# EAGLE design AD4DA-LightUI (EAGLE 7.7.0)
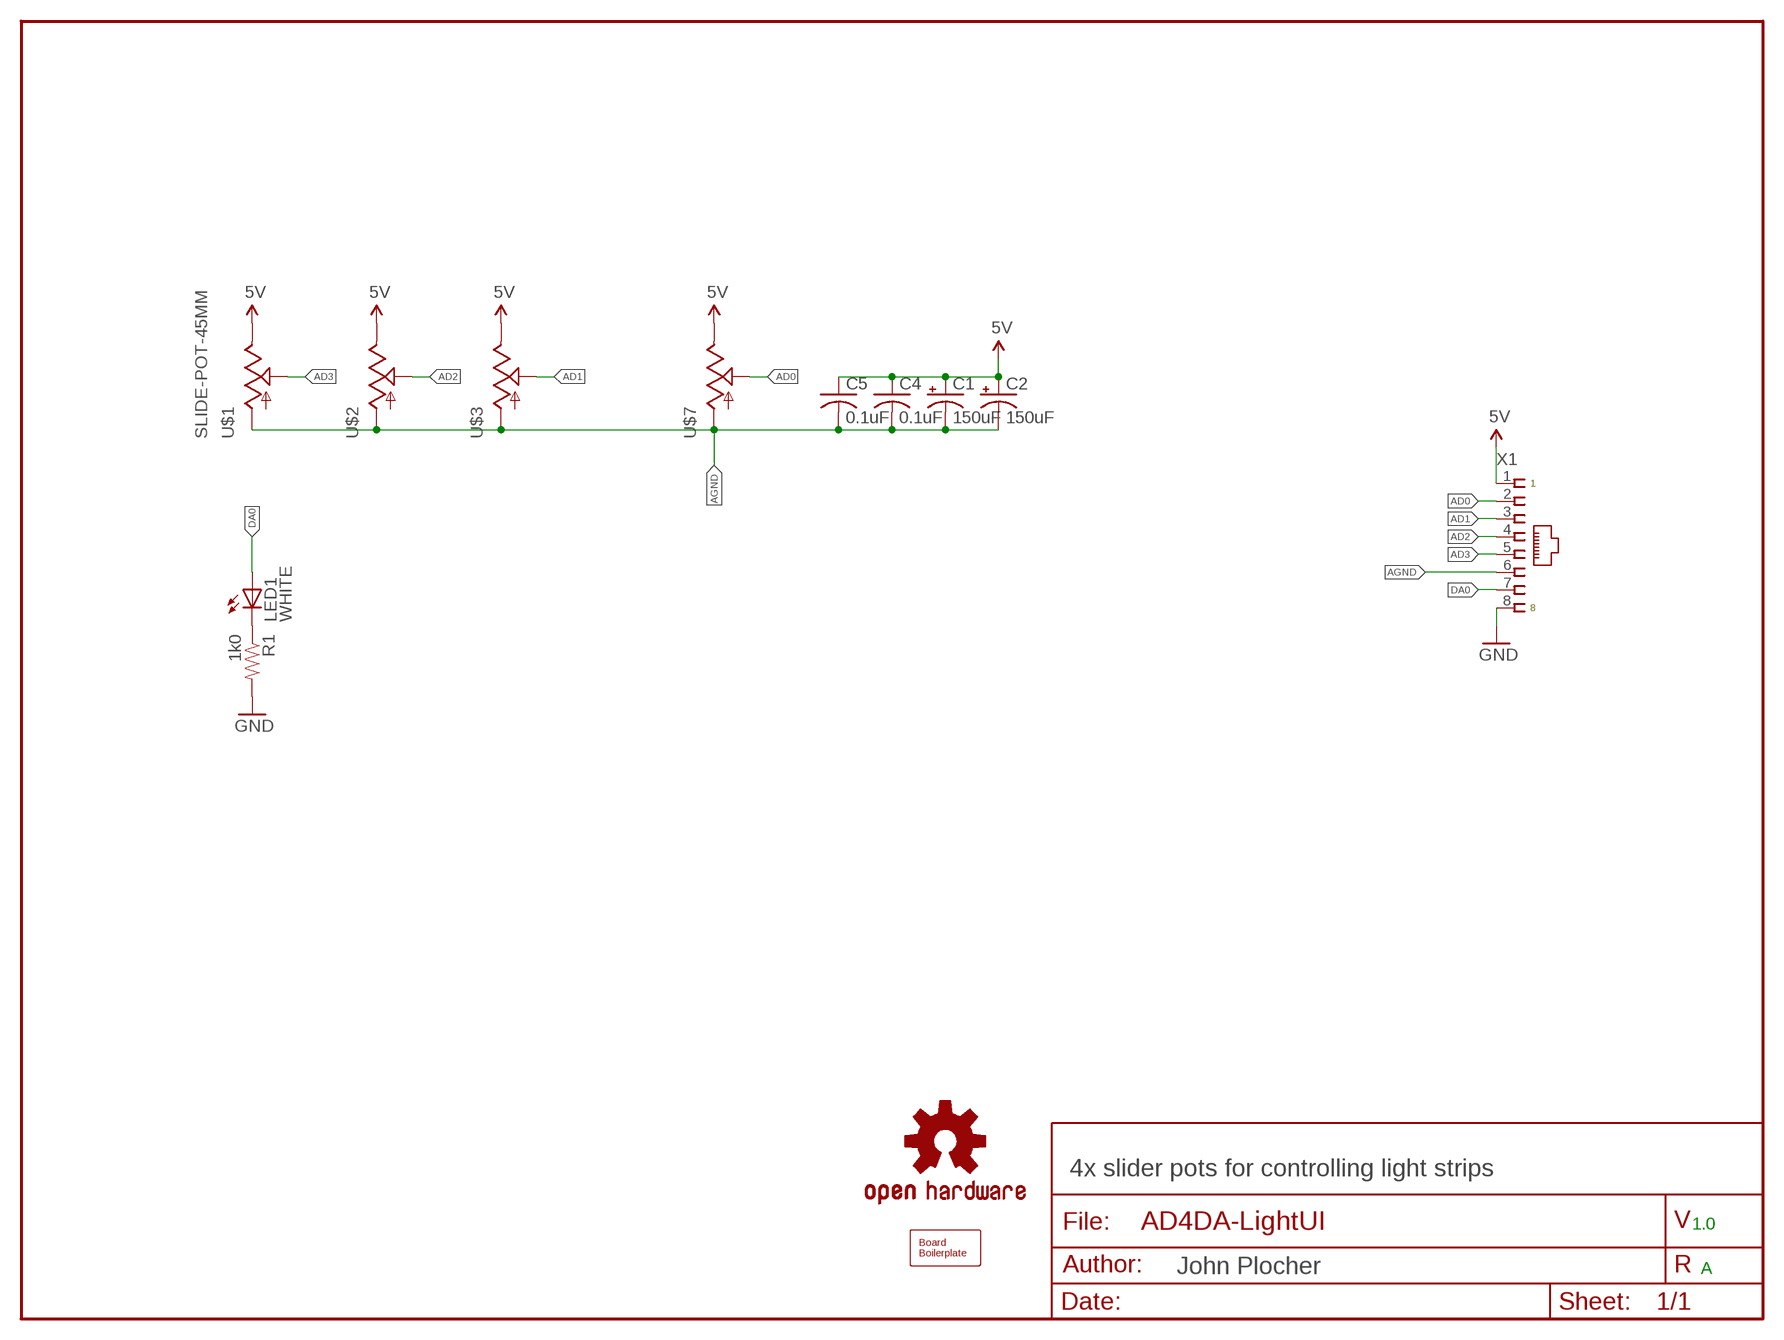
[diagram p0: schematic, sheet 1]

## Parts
C1  150uF  CAP-POLPTH-5MM  [E5-10.5]
C2  150uF  CAP-POLPTH-5MM  [E5-10.5]
C4  0.1uF  CAPPTH1  [C050-024X044]
C5  0.1uF  CAPPTH1  [C050-024X044]
LED1  WHITE  LEDLED5MM  [LED5MM]
LOGO1  DOC-OSHW-LOGO-L  [OSHW-LOGO-L]
R1  1k0  RPTH03  [AXIAL-0.3-RES]
U$1  SLIDE-POT-45MM  R-SLIDE-POT  [SLIDER-45MM-LARGE]
U$2  R-SLIDE-POT  [SLIDER-45MM-LARGE]
U$3  R-SLIDE-POT  [SLIDER-45MM-LARGE]
U$7  R-SLIDE-POT  [SLIDER-45MM-LARGE]
U$9  BOARD80X100  [BOARD-DINRAIL-3.17INX10CM]
X1  CONNECTOR-RJ45-FRONT  [RJ45-NO-SHIELD]

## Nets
5V: C1.+ C2.+ C4.1 C5.1 U$1.E U$2.E U$3.E U$7.E X1.1
AD0: U$7.S X1.2
AD1: U$3.S X1.3
AD2: U$2.S X1.4
AD3: U$1.S X1.5
AGND: C1.- C2.- C4.2 C5.2 U$1.A U$2.A U$3.A U$7.A X1.6
DA0: LED1.A X1.7
GND: R1.P$2 X1.8
N$2: LED1.K(C) R1.P$1
Unconnected: U$1.AGND@0(AGND) U$2.AGND@0(AGND) U$3.AGND@0(AGND) U$7.AGND@0(AGND)

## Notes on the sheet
- 4x slider pots for controlling light strips
- 1.0
- A

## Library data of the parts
C1 C2 = SPCoast:CAP-POL*
C4 C5 = SPCoast:CAP*
LED1 = SPCoast:LED*
LOGO1 = SPCoast:DOC-OSHW-LOGO-: Open Source Hardware Logo
R1 = SPCoast:R*: Resistor
U$1-U$3 U$7 = SPCoast:R-SLIDE-POT: Slide-type potentiometer- COM-9119
U$9 = SPCoast:BOARD
X1 = SPCoast:CONNECTOR-RJ45: Tyco CORCOM Modular RJ Jacks No Shield; AMP: 520151-4; OPL: none

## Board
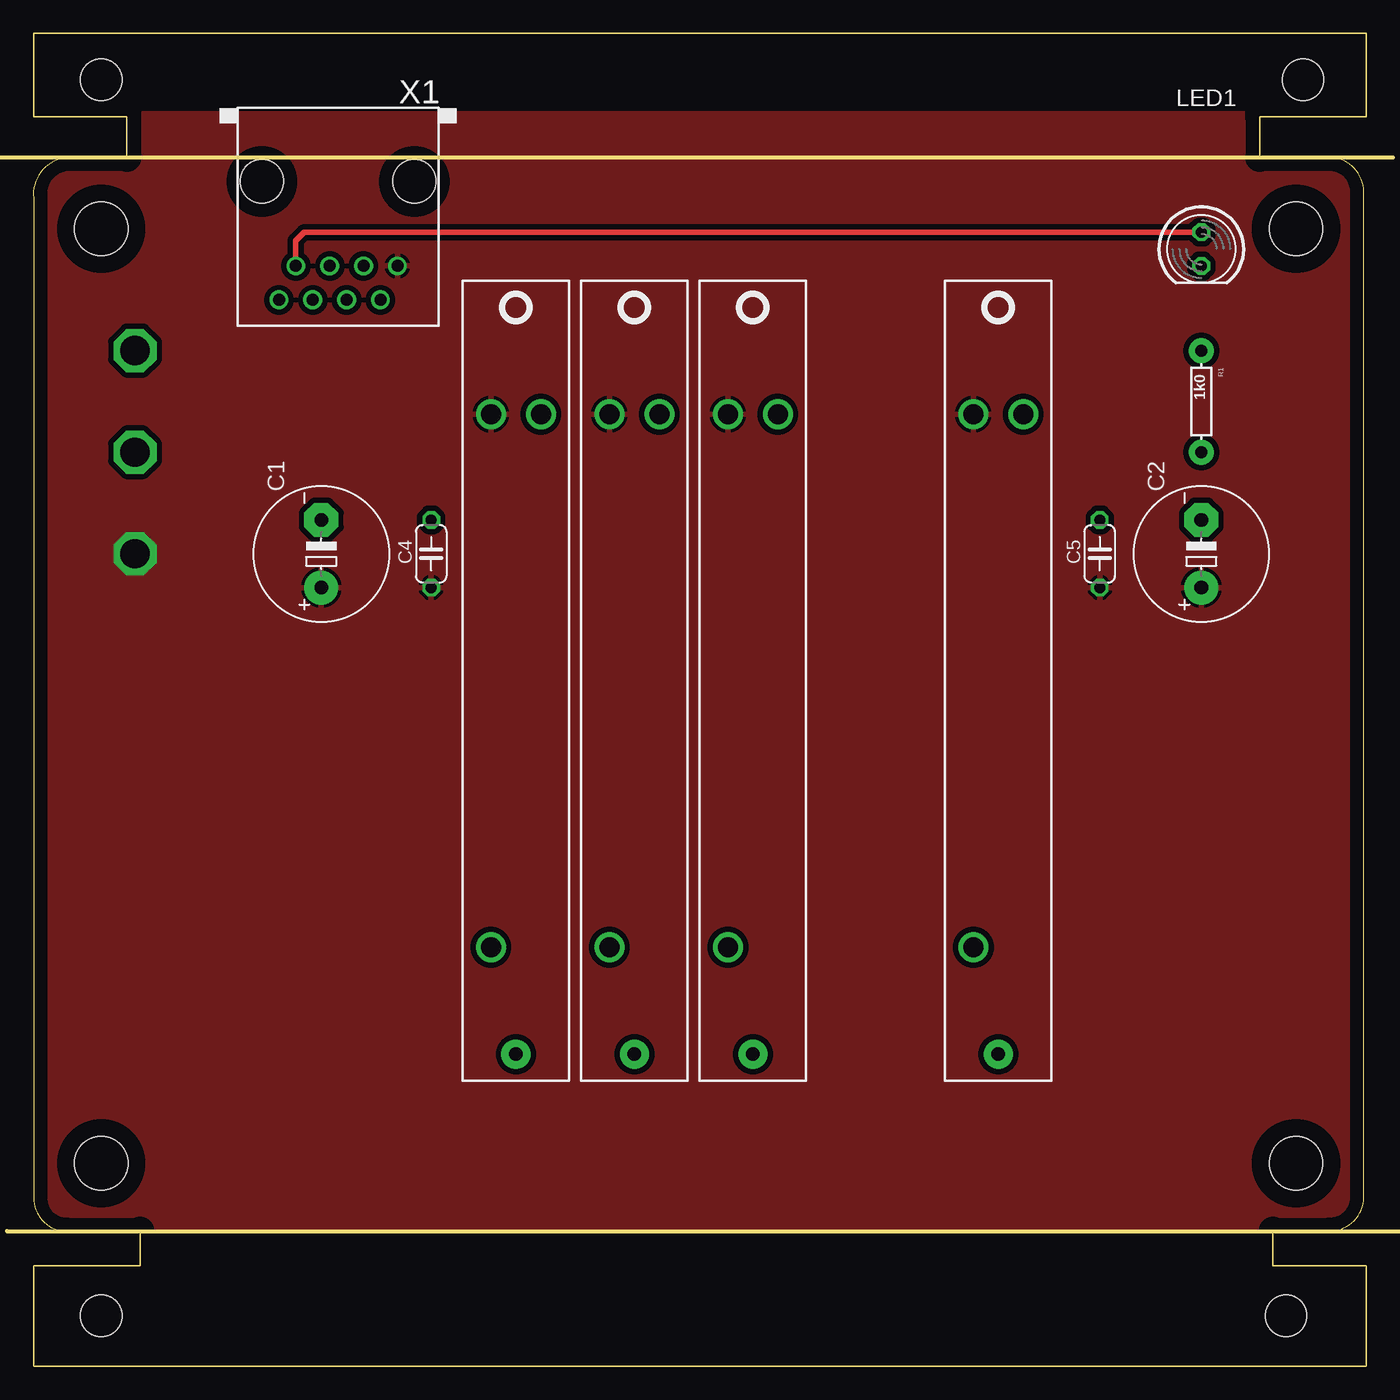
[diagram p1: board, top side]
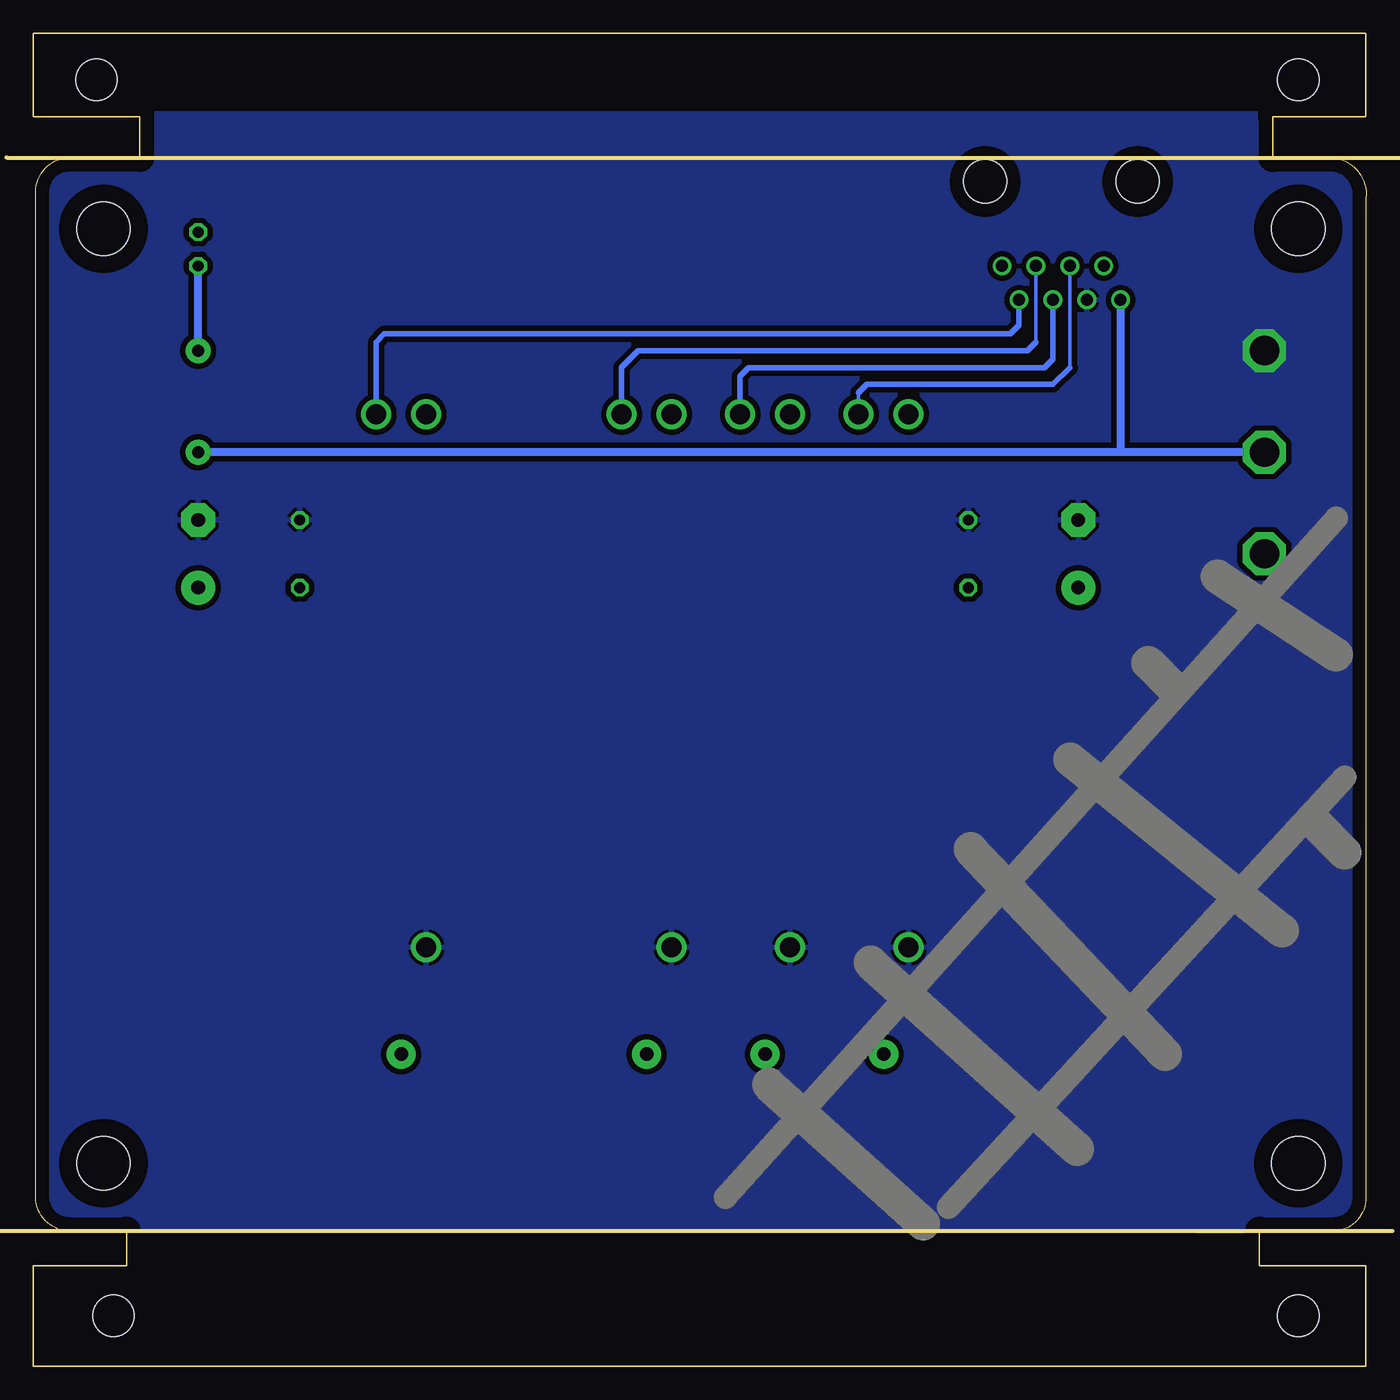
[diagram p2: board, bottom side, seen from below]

Size 100.01 x 100 mm. Coordinates in mm from the lower left corner, seen from the top.
Copper layers (1*16): Top 0.035mm / dielectric 1.5mm / Bottom 0.035mm
Design rules "default": minimum track width 10mil, minimum drill 0.6mm, track to track 8mil, track to pad 8mil, pad to pad 8mil, via to via 8mil, smd to smd 8mil, copper to edge 40mil, drill to drill 8mil, minimum pad ring 10mil, minimum via ring 8mil, stop-mask expansion 4mil, vias tented up to drill 0mil, thermal gap 10mil

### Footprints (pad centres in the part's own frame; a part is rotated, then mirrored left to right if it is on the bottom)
E5-10.5 = drill 1.016 pad 2.54: + -2.54,0 | drill 1.016 pad 2.54 octagon: - 2.54,0
C050-024X044 = drill 0.813 octagon: 1 -2.54,0; 2 2.54,0
LED5MM = drill 0.813 octagon: A -1.27,0; K 1.27,0
AXIAL-0.3-RES = drill 0.9 pad 1.88: P$1 -3.81,0; P$2 3.81,0
SLIDER-45MM-LARGE = drill 1.5: A 20,-1.875; E -20,-1.875; S -20,1.875 | drill 1 pad 2.184: AGND@0 28,0
BOARD-DINRAIL-3.17INX10CM = hole 4: 94.742,15.24; 5.08,85.344; 94.742,85.344; 5.08,15.24 | hole 3.1: 5.08,96.52; 95.25,96.52; 5.08,3.81; 93.98,3.81
RJ45-NO-SHIELD = drill 0.9 pad 1.4: 1 -4.445,6.35; 2 -3.175,8.89; 3 -1.905,6.35; 4 -0.635,8.89; 5 0.635,6.35; 6 1.905,8.89; 7 3.175,6.35; 8 4.445,8.89 | hole 3.251: -5.715,0; 5.715,0

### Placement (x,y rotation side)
C1  21.6,60.96 90 top
C2  87.64,60.96 90 top
C4  29.86,60.96 90 top
C5  80.02,60.96 90 top
LED1  87.64,83.82 270 top
LOGO1  5.09,85.09 0 top
R1  87.64,72.39 270 top
U$1  36.21,51.44 270 top
U$2  45.1,51.44 270 top
U$3  53.99,51.44 270 top
U$7  72.4,51.44 270 top
U$9  0.01,0 0 top
X1  22.87,88.9 180 top

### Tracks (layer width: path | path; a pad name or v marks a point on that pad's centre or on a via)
5V  (via drill 2.2)
  other vias: 7.63,60.96
  pour Top (isolate 0.406): 0.01,93.98 102.55,93.98 102.55,10.43 0.01,10.16
AD0
  Bottom 0.254: 74.31,76.83 74.28,76.81
  Bottom 0.406: X1.2 26.05,78.11 26.68,77.47 73.67,77.47 74.31,76.83 | 74.28,76.81 U$7.S
AD1
  Bottom 0.254: X1.3 24.78,76.83
  Bottom 0.406: 24.78,76.83 25.41,76.2 54.62,76.2 55.86,74.96 U$3.S
AD2
  Bottom 0.406: X1.4 23.51,75.56 24.14,74.93 46.37,74.93 47,74.3 46.97,72.36 U$2.S
AD3
  Bottom 0.254: X1.5 22.24,74.93 | 38.11,73.03 38.11,72.39 | 38.08,71.15 U$1.S
  Bottom 0.406: 22.24,74.93 23.51,73.66 37.48,73.66 38.11,73.03 | 38.11,72.39 38.08,71.15
AGND  (via drill 2.2)
  other vias: 7.63,76.2
  pour Bottom (isolate 0.406): 0.01,93.98 102.09,93.98 102.09,10.43 0.01,10.16
DA0
  Top 0.406: X1.7 19.7,84.45 20.33,85.09 LED1.A
GND  (via drill 2.2)
  Bottom 0.61: X1.8 18.43,68.58 | 18.43,68.58 R1.P$2 | v7.63,68.58 18.43,68.58
N$2
  Bottom 0.61: R1.P$1 LED1.K

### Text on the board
tDocu: v1.0 | D/A out | DA0 | R G B | White | OSHW | Agnd | DA0 | AD3 | AD2 | AD1 | AD0 | +5 | AD3 | AD2 | AD1 | AD0 | Dgnd | Agnd | Dgnd | +5 | LightUI | 2014-10 A
bDocu: Made in the PCR, Coast Division, NMRA | LightUI | Solder Side | Go Bears! | Model Railroading is fun! | www . SPCoast . com

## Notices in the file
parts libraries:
SparkFun-Aesthetics: Licensing: CC v3.0 Share-Alike You are welcome to use this library for commercial purposes.
SPCoast: http://freedomdefined.org/OSHW Creative Commons - Attribution - ShareAlike 3.0
